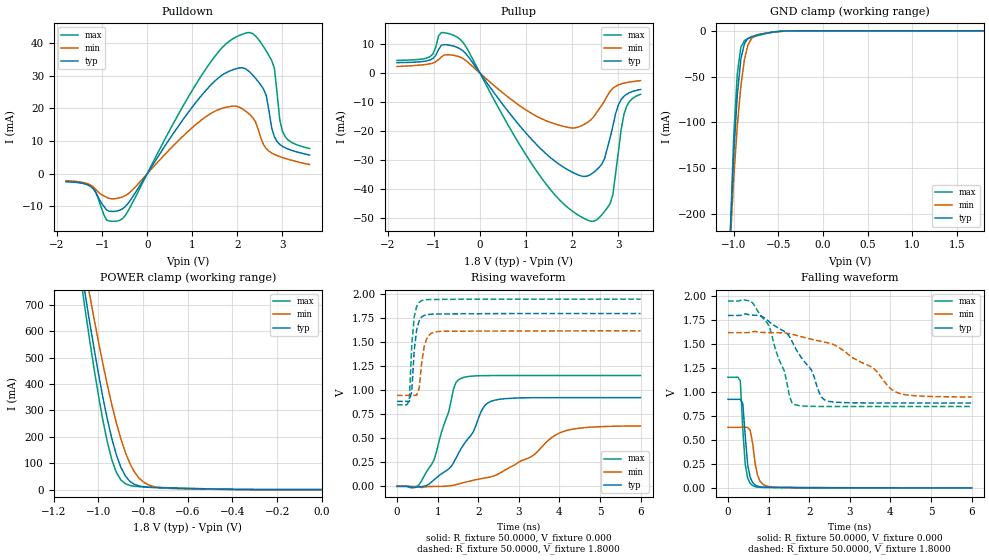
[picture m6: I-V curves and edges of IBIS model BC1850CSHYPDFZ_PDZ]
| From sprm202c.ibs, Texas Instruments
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|   Model BC1850CSHYPDFZ_PDZ
[Model]   BC1850CSHYPDFZ_PDZ
Model_type   I/O
Polarity   Non-Inverting
Enable   Active-Low
Vinl =   0.8500V
Vinh =   0.9800V
Vmeas =   0.9000V
Cref =  15.0000pF
Rref = 100.0000M
Vref =  0.000V
C_comp   1.3000pF   1.4700pF   1.1000pF
[Model Spec]
|   typ   min   max
Vinh   0.98V   0.86V   1.1V
Vinl   0.85V   0.70V   0.91V
[Temperature Range]   25.0000   0.1250k   -40.0000
[Voltage Range]   1.8000V   1.6200V   1.9500V
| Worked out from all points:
|   slope of the pulldown table from 0 to 0.27 V, typ, clamps not added: 46 ohm
|   slope of the pullup table from 0 to 0.27 V, typ, clamps not added: 44.9 ohm
|   GND clamp passes 1 mA (typ) near -0.52 V on its own axis
|   POWER clamp passes 1 mA (typ) near -0.40 V on its own axis
|   rising waveform, R_fixture 50.0000, V_fixture 0.000: 20-80 % time 751ps typ, 1.31ns min, 494ps max; typ from 0 V to 0.924 V
|   rising waveform, R_fixture 50.0000, V_fixture 1.8000: 20-80 % time 106ps typ, 132ps min, 95.3ps max; typ from 0.885 V to 1.8 V
|   falling waveform, R_fixture 50.0000, V_fixture 0.000: 20-80 % time 121ps typ, 143ps min, 103ps max; typ from 0.924 V to 0 V
|   falling waveform, R_fixture 50.0000, V_fixture 1.8000: 20-80 % time 745ps typ, 1.25ns min, 512ps max; typ from 1.8 V to 0.885 V
[Pulldown]
| voltage   I(typ)   I(min)   I(max)
-1.8V     -2.432mA   -2.13mA    -2.324mA
-1.2V     -4.535mA   -3.994mA   -4.328mA
-900mV    -11.04mA   -7.186mA   -14.12mA
-540mV    -10.64mA   -7.052mA   -13.61mA
1.32V     25.76mA    17.6mA     32.41mA
2.22V     31.69mA    18.71mA    43.1mA
2.58V     25.85mA    8.892mA    38.8mA
2.76V     14.03mA    6.343mA    34.57mA
2.82V     11.26mA    5.911mA    32.25mA
2.94V     8.959mA    5.237mA    16.41mA
3.06V     7.924mA    4.688mA    11.3mA
3.6V      5.706mA    2.822mA    7.711mA
[Pullup]
| voltage   I(typ)   I(min)   I(max)
-1.8V     3.669mA    2.32mA     4.446mA
-1.08V    4.598mA    3.276mA    5.779mA
-840mV    9.631mA    5.639mA    14.06mA
-420mV    8.322mA    5.5mA      11.54mA
1.32V     -26.18mA   -15.62mA   -35.92mA
1.98V     -34.04mA   -18.91mA   -47.41mA
2.4V      -34.97mA   -16.12mA   -51.17mA
2.64V     -31.45mA   -11.07mA   -48.94mA
2.82V     -22.35mA   -6.261mA   -45.06mA
2.88V     -18.23mA   -5.221mA   -41.92mA
3.12V     -7.968mA   -3.432mA   -14.2mA
3.48V     -5.617mA   -2.562mA   -7.289mA
[GND_clamp]
| voltage   I(typ)   I(min)   I(max)
-1.8V     -5.333A    -4.658A    -5.852A
-1.04V    -226.9mA   -235.1mA   -226.4mA
-1V       -135.8mA   -161.8mA   -116.3mA
-960mV    -70.57mA   -104.3mA   -47.27mA
-920mV    -30.97mA   -60.68mA   -18.06mA
-880mV    -13.88mA   -31.39mA   -10.61mA
-840mV    -8.324mA   -15.39mA   -8.431mA
-800mV    -6.322mA   -8.275mA   -7.135mA
-720mV    -4.296mA   -3.956mA   -4.93mA
-600mV    -2.054mA   -1.978mA   -2.087mA
-360mV    -85.5uA    -157.2uA   -38.41uA
1.8V      8.754nA    3.628uA    12.16nA
[POWER_clamp]
| voltage   I(typ)   I(min)   I(max)
-1.8V     5.299A     4.889A     5.644A
-1.08V    850.2mA    929.8mA    802mA
-1.06V    742mA      833.5mA    683.6mA
-1.04V    636.8mA    739.4mA    568.9mA
-1V       438.8mA    559.8mA    355.8mA
-960mV    265.5mA    395.4mA    178.9mA
-940mV    192.5mA    321mA      112.5mA
-920mV    131.7mA    253.1mA    65.29mA
-880mV    52.26mA    141.7mA    22.44mA
-820mV    14.13mA    45.17mA    11.23mA
-740mV    7.184mA    9.386mA    8.475mA
0V        8.78nA     22.3nA     13.47nA
[Ramp]
| variable   typ   min   max
dV/dt_r   0.5546/0.7488n   0.3788/1.3695n   0.6926/0.4977n
dV/dt_f   0.5489/0.7449n   0.4037/1.3068n   0.6605/0.5166n
R_load = 50.0000
[Rising Waveform]
R_fixture = 50.0000
V_fixture = 0.000
V_fixture_min = 0.000
V_fixture_max = 0.000
| time   V(typ)   V(min)   V(max)
0s        534nV      1.078uV    250.2nV
484.8ps   -6.765mV   -2.211mV   -1.967mV
848.5ps   43.96mV    -1.404mV   226.8mV
1.273ns   180.6mV    4.053mV    774.6mV
1.394ns   246.5mV    12.64mV    1.016V
1.576ns   390.3mV    31.59mV    1.123V
2.121ns   817.3mV    83.68mV    1.153V
2.364ns   892.6mV    105.3mV    1.154V
4.121ns   923.8mV    574.3mV    1.154V
6ns       924.2mV    629mV      1.154V
[Rising Waveform]
R_fixture = 50.0000
V_fixture = 1.8000
V_fixture_min = 1.6200
V_fixture_max = 1.9500
| time   V(typ)   V(min)   V(max)
0s        885.2mV    946.9mV    849.1mV
303ps     884.3mV    947.4mV    894.1mV
363.6ps   988.8mV    947mV      1.475V
424.2ps   1.416V     946.6mV    1.766V
484.8ps   1.632V     950.1mV    1.875V
545.5ps   1.723V     1.022V     1.916V
606.1ps   1.762V     1.276V     1.935V
727.3ps   1.788V     1.535V     1.945V
969.7ps   1.795V     1.61V      1.946V
6ns       1.8V       1.62V      1.95V
[Falling Waveform]
R_fixture = 50.0000
V_fixture = 0.000
V_fixture_min = 0.000
V_fixture_max = 0.000
| time   V(typ)   V(min)   V(max)
0s        924.3mV    631.6mV    1.154V
303ps     924.8mV    631.6mV    1.118V
363.6ps   880.8mV    631.6mV    617.1mV
424.2ps   542.8mV    631.9mV    244.3mV
484.8ps   237.7mV    631.7mV    103mV
545.5ps   110.7mV    600.8mV    47.75mV
606.1ps   55.48mV    465.5mV    24.17mV
727.3ps   17.55mV    130.6mV    7.428mV
969.7ps   6.01mV     16.33mV    3.952mV
6ns       52.28uV    382.6uV    299.1nV
[Falling Waveform]
R_fixture = 50.0000
V_fixture = 1.8000
V_fixture_min = 1.6200
V_fixture_max = 1.9500
| time   V(typ)   V(min)   V(max)
0s        1.8V       1.62V      1.95V
545.5ps   1.805V     1.623V     1.951V
969.7ps   1.75V      1.621V     1.722V
1.394ns   1.632V     1.617V     1.214V
1.515ns   1.578V     1.609V     955.2mV
1.636ns   1.479V     1.597V     869.9mV
2.424ns   909.4mV    1.517V     849.5mV
3.576ns   886.1mV    1.251V     849.1mV
4.182ns   885.6mV    991.9mV    849.1mV
6ns       885.3mV    948.8mV    849.1mV
